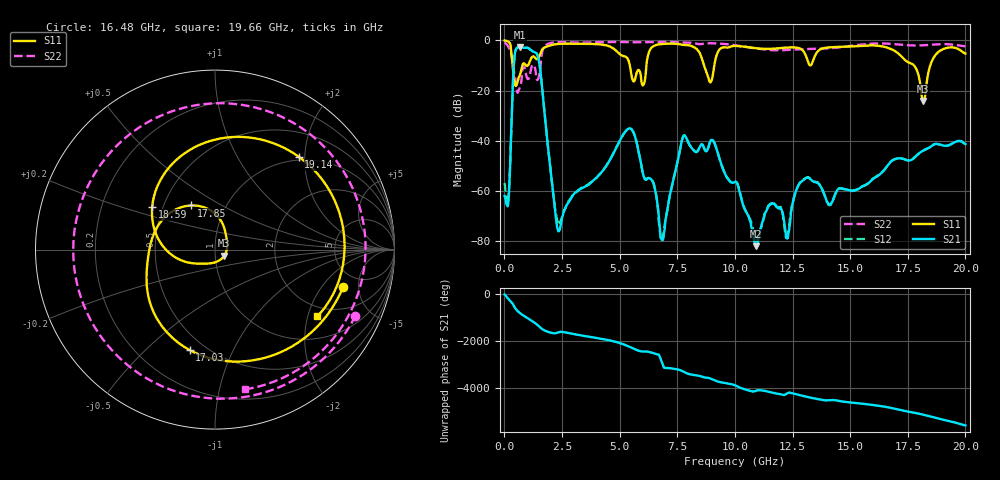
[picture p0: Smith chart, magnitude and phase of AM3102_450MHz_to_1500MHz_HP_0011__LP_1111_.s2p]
!Agilent Technologies,E8364B,MY43040894,A.07.50.67
!Agilent E8364B: A.07.50.67
!Date: Thursday, January 11, 2018 05:34:12
!Correction: S11(Full 2 Port(1,2))
!S21(Full 2 Port(1,2))
!S12(Full 2 Port(1,2))
!S22(Full 2 Port(1,2))
!S2P File: Measurements: S11, S21, S12, S22:
# Hz S  dB  R 50
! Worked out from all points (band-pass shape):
!   1601 points, 10 MHz to 20 GHz, reference 50 ohm
!   highest |S21| = -2.70 dB at 659.7 MHz (marker M1); lowest = -81.9 dB at 10.9 GHz (marker M2)
!   |S21| within 3 dB of the highest: 449.2 MHz to 1.427 GHz (978.1 MHz wide, 104 % of centre)
!   lowest |S11| = -24.2 dB at 18.18 GHz (marker M3), VSWR 1.13, Z = 55.3 - j3.77 ohm
!   |S11| at or under -10 dB: 5.441 GHz to 6.16 GHz (719.5 MHz wide, 12.4 % of centre); 8.664 GHz to 9.108 GHz (443.9 MHz wide, 5 % of centre); 17.77 GHz to 18.47 GHz (705.7 MHz wide, 3.89 % of centre)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
!   |S22| runs from -20.8 to -0.6 dB; largest |S21 - S12| = 0.004
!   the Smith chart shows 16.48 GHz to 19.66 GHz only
!   S11 on the Smith chart (normalised r, x): 16.48 GHz: 3.56, -3.31; 17.03 GHz: 0.41, -0.69; 17.85 GHz: 0.69, +0.37; 18.59 GHz: 0.44, +0.25; 19.14 GHz: 0.93, +1.87; 19.66 GHz: 1.66, -2.30
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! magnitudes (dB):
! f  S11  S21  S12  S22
! 10 MHz  -0.1  -61.9  -56.8  -0.8
! 172.4 MHz  -0.6  -64.1  -63.7  -2.6
! 434.8 MHz  -16.2  -6.9  -6.9  -13.5
! 659.7 MHz  -14.1  -2.7  -2.7  -19.1
! 1.484 GHz  -6.9  -7.5  -7.5  -14.9
! 2.334 GHz  -1.5  -75.9  -73.1  -0.7
! 3.346 GHz  -1.4  -58.9  -58.6  -0.9
! 5.457 GHz  -10.8  -35.1  -35.1  -0.7
! 6.682 GHz  -1.6  -68.1  -70.3  -0.7
! 7.806 GHz  -1.9  -37.8  -37.8  -0.8
! 10.01 GHz  -2.2  -56.3  -56.3  -2.0
! 10.9 GHz  -3.1  -81.9  -79.9  -3.2
! 13.34 GHz  -9.3  -55.8  -55.7  -3.4
! 16.48 GHz  -2.6  -51.6  -51.6  -1.3
! 16.68 GHz  -3.1  -49.2  -49.2  -1.4
! 17.03 GHz  -4.8  -47.1  -47.0  -1.6
! 17.85 GHz  -11.1  -46.1  -46.1  -2.0
! 18.18 GHz  -24.2  -43.8  -43.9  -2.0
! 18.59 GHz  -7.5  -41.7  -41.7  -1.7
! 19.14 GHz  -3.1  -42.0  -42.0  -1.5
! 19.66 GHz  -3.3  -40.1  -40.1  -2.0
! 20 GHz  -5.3  -41.3  -41.4  -2.4
